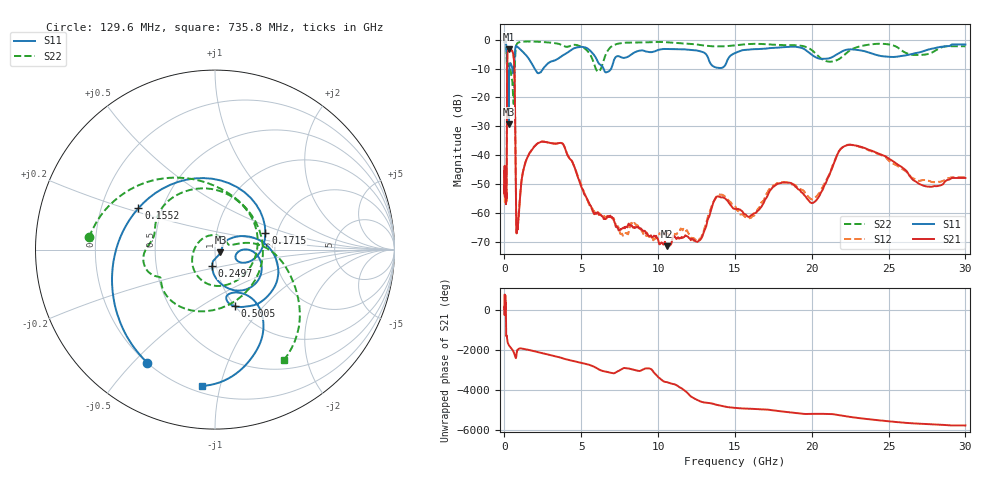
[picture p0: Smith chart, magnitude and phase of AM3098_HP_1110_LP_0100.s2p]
! Date/Time: Thu, Feb 28, 2019 8:46 AM
! Network Analyzer: Agilent Technologies E8364B Rev: A.07.50.67
! Sweep from 0.010 to 30.000 GHz, 1601 Points, Sweep Type: LOG
! Power Supply: 5.023 V, 0.002 A
# Hz S DB R 50
!freq MagS11 AngS11 MagS21 AngS21 MagS12 AngS12 MagS22 AngS22
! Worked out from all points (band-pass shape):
!   1601 points, 10 MHz to 30 GHz, reference 50 ohm
!   highest |S21| = -3.40 dB at 285.8 MHz (marker M1); lowest = -71.5 dB at 10.59 GHz (marker M2)
!   |S21| within 3 dB of the highest: 183.3 MHz to 606.9 MHz (423.7 MHz wide, 107 % of centre)
!   lowest |S11| = -29.4 dB at 263.8 MHz (marker M3), VSWR 1.07, Z = 53.1 - j1.56 ohm
!   |S11| at or under -10 dB: 170.1 MHz to 319.8 MHz (149.7 MHz wide, 61.1 % of centre); 1.959 GHz to 2.528 GHz (568.9 MHz wide, 25.4 % of centre); 6.446 GHz to 6.947 GHz (500.6 MHz wide, 7.48 % of centre)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
!   |S22| runs from -22.3 to -0.5 dB; largest |S21 - S12| = 0.01
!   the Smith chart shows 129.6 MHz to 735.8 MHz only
!   S11 on the Smith chart (normalised r, x): 129.6 MHz: 0.20, -0.55; 155.2 MHz: 0.37, +0.22; 171.5 MHz: 1.73, +0.35; 249.7 MHz: 0.95, -0.18; 500.5 MHz: 1.00, -0.71; 735.8 MHz: 0.24, -0.88
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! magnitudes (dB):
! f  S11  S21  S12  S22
! 10 MHz  -0.3  -45.5  -47.2  -0.5
! 38.04 MHz  -0.3  -51.4  -50.5  -0.6
! 129.6 MHz  -2.7  -53.6  -55.1  -3.0
! 144.7 MHz  -4.3  -49.5  -50.3  -5.7
! 155.2 MHz  -6.3  -34.3  -34.2  -10.5
! 171.5 MHz  -10.6  -11.5  -11.4  -8.7
! 249.7 MHz  -20.6  -3.6  -3.5  -8.8
! 263.8 MHz  -29.4  -3.5  -3.4  -9.1
! 285.8 MHz  -16.5  -3.4  -3.3  -9.0
! 500.5 MHz  -9.5  -3.9  -3.9  -14.0
! 550.5 MHz  -11.4  -4.6  -4.5  -19.1
! 655.8 MHz  -6.0  -12.1  -12.1  -13.0
! 735.8 MHz  -2.3  -52.3  -50.5  -2.8
! 821.5 MHz  -2.4  -65.0  -64.0  -1.4
! 2.084 GHz  -11.2  -36.3  -36.3  -0.7
! 3.798 GHz  -5.5  -36.1  -36.0  -2.0
! 6.11 GHz  -8.0  -59.9  -60.2  -11.1
! 7.926 GHz  -6.2  -64.9  -67.0  -1.0
! 10.59 GHz  -3.3  -71.5  -67.0  -0.9
! 20.1 GHz  -5.6  -56.5  -55.2  -4.1
! 22.67 GHz  -3.4  -36.5  -36.6  -3.2
! 30 GHz  -1.7  -47.9  -47.7  -2.3
